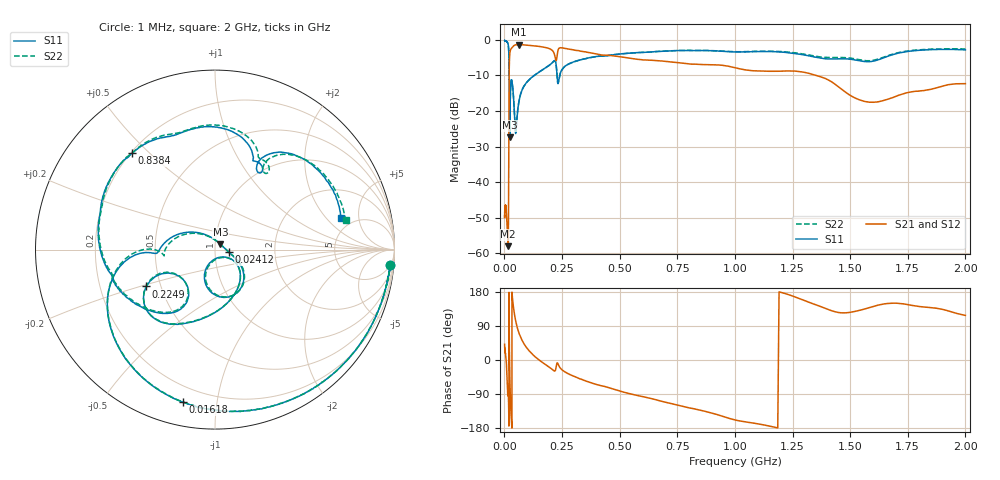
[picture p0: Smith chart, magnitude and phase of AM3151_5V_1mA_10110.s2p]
! Date/Time: Fri Jun 26 10:57:16 2020
! Network Analyzer:  Rev:
! Sweep from 1000000.0 to 2000000000.0, 1601 Points ! Power Supply: 0 V, 0 A
# HZ S DB R 50
!freq MagS11 AngS11 MagS21 AngS21 MagS12 AngS12 MagS22 AngS22
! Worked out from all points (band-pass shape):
!   1601 points, 1 MHz to 2 GHz, reference 50 ohm
!   highest |S21| = -1.31 dB at 61.77 MHz (marker M1); lowest = -58.0 dB at 16.41 MHz (marker M2)
!   |S21| within 3 dB of the highest: 23 MHz to 218.1 MHz (195.1 MHz wide, 162 % of centre); 229.1 MHz to 445.5 MHz (216.4 MHz wide, 64.2 % of centre)
!   lowest |S11| = -27.4 dB at 23.22 MHz (marker M3), VSWR 1.09, Z = 53 + j3.18 ohm
!   |S11| at or under -10 dB: 20.72 MHz to 129.3 MHz (108.6 MHz wide, 145 % of centre); 228.5 MHz to 240.1 MHz (11.61 MHz wide, 4.96 % of centre)
!   |S22| runs from -27.4 to -0.2 dB; largest |S21 - S12| = 0.0058
!   S11 on the Smith chart (normalised r, x): 1 MHz: 4, -21; 16.18 MHz: 0.12, -0.81; 24.12 MHz: 1.16, -0.03; 224.9 MHz: 0.41, -0.21; 838.4 MHz: 0.21, +0.44; 2 GHz: 3.95, +2.93
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1000000  -0.17 -5.2  -49.45 41.5  -50.10 39.2  -0.17 -5.2
3555161  -0.24 -17.6  -46.71 20.2  -46.72 19.9  -0.24 -17.5
1.263916e7  -0.63 -69.6  -53.51 -65.8  -53.55 -66.4  -0.65 -69.8
1.618087e7  -1.22 -101.8  -58.00 -91.7  -57.60 -90.5  -1.26 -102.7
1.641312e7  -1.29 -104.6  -58.04 -86.9  -57.88 -86.5  -1.32 -105.5
1.779362e7  -1.90 -124.5  -51.65 -98.0  -51.53 -98.3  -1.99 -126.2
2.051914e7  -9.70 -176.3  -10.24 108.8  -10.23 108.8  -10.89 -173.0
2.151743e7  -12.80 158.9  -6.66 41.0  -6.67 41.0  -13.18 161.3
2.32167e7  -27.39 44.4  -4.12 -31.5  -4.12 -31.5  -27.35 40.8
2.411603e7  -22.22 -10.1  -3.54 -58.6  -3.54 -58.6  -22.17 -10.1
2.65197e7  -14.29 -36.6  -2.81 -110.0  -2.82 -110.0  -14.37 -35.0
3.116846e7  -11.24 -74.5  -2.32 -167.0  -2.33 -167.0  -11.27 -72.6
4.493426e7  -22.50 -109.9  -1.47 116.4  -1.48 116.4  -22.27 -106.5
4.964819e7  -26.25 -64.4  -1.38 101.4  -1.39 101.3  -25.63 -63.5
6.177434e7  -17.89 -31.5  -1.31 73.9  -1.32 73.8  -17.81 -31.9
1.589914e8  -8.66 -94.8  -1.91 -3.8  -1.91 -3.8  -8.69 -95.0
2.248969e8  -7.24 -151.8  -5.83 -17.4  -5.84 -17.4  -7.17 -151.8
5.652395e8  -3.64 171.4  -5.36 -92.0  -5.33 -92.0  -3.64 169.4
8.384428e8  -3.00 130.6  -6.88 -131.0  -6.83 -130.9  -2.97 128.3
1.304205e9  -4.28 72.0  -9.17 156.3  -9.10 156.2  -4.04 69.7
1.584655e9  -6.13 61.2  -17.54 138.6  -17.56 138.3  -5.86 57.6
2e9  -2.82 14.2  -12.32 117.7  -12.47 116.8  -2.55 12.6
